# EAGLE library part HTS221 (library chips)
Capacitive humidity sensor 2mmx2mm
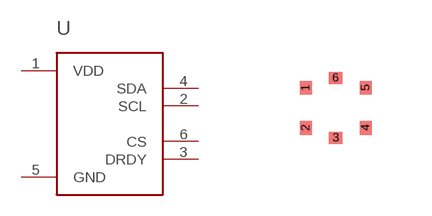
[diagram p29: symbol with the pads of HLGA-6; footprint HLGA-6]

Designator prefix -

## HTS221  [HLGA-6]
1  VDD
2  SCL
3  DRDY
4  SDA
5  GND
6  CS

## Footprint HLGA-6 (pad centres in mm)
smd 0.3 x 0.35: 1 -0.75,0.5; 2 -0.75,-0.5; 4 0.75,-0.5; 5 0.75,0.5
smd 0.35 x 0.3: 3 0,-0.75; 6 0,0.75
